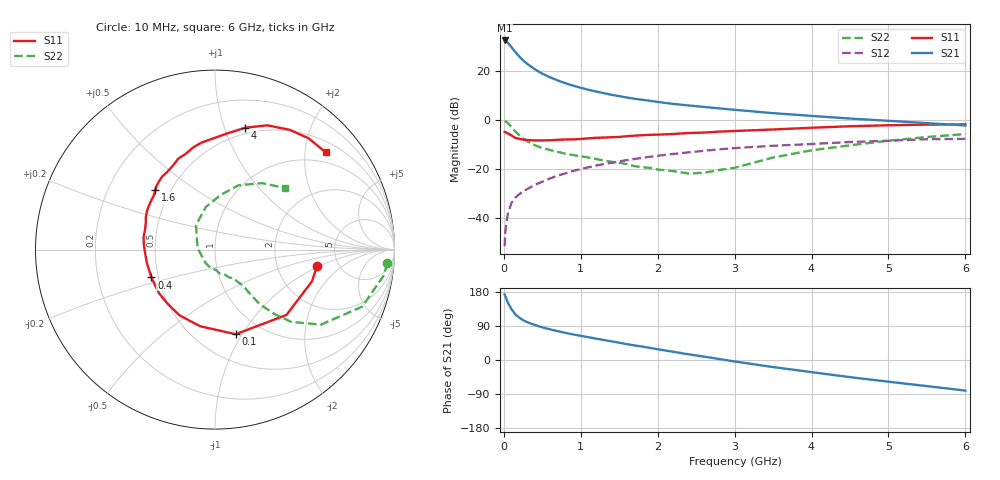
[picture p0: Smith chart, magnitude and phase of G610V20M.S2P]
! SIEMENS Small Signal Semiconductors
! BFG193
! Si NPN RF Bipolar Junction Transistor in SOT223
! VCE = 10 V  IC = 20 mA
! Common Emitter S-Parameters:  August  1996
# GHz  S  MA  R  50
!  f  S11  S21  S12  S22
! GHz  MAG  ANG  MAG  ANG  MAG  ANG  MAG  ANG
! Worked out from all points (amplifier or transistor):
!   36 points, 10 MHz to 6 GHz, reference 50 ohm
!   highest |S21| = 32.5 dB at 10 MHz (marker M1)
!   |S21| within 3 dB of that: start of sweep to 106.1 MHz
!   unconditionally stable (mu >= 1): 743.1 MHz to 2.596 GHz
!   at 250 MHz: K = 0.72, MSG = 26.7 dB, |S12| = -29.1 dB
!   at 1.4 GHz: K = 1.05, MAG = 12.5 dB, |S12| = -17.4 dB
!   at 6 GHz: K = 0.88, MSG = 2.7 dB, |S12| = -7.6 dB
!   S11 on the Smith chart (normalised r, x): 10 MHz: 3.45, -0.92; 100 MHz: 0.76, -0.94; 400 MHz: 0.46, -0.17; 1.6 GHz: 0.41, +0.35; 4 GHz: 0.44, +1.18; 6 GHz: 0.74, +2.46
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0.01  0.5756 -8.9  42.12 173.3  0.0027 89.0  0.9638 -4.5
0.02  0.5687 -18.1  41.56 168.5  0.0054 82.9  0.9491 -9.0
0.05  0.5395 -42.5  38 152.2  0.012 73.4  0.8792 -21.2
0.1  0.4852 -76.3  30.69 134.1  0.0207 64.0  0.7235 -35.3
0.15  0.435 -101.0  24.26 120.1  0.0264 58.6  0.5847 -43.5
0.2  0.4162 -118.4  19.89 111.9  0.0309 58.4  0.4931 -47.1
0.25  0.4007 -131.7  16.58 105.1  0.0352 58.0  0.4214 -49.5
0.3  0.3951 -142.4  14.2 100.2  0.0392 59.1  0.3755 -50.9
0.4  0.3868 -156.4  10.97 92.7  0.0476 59.6  0.3094 -51.7
0.5  0.3868 -168.5  8.856 86.1  0.0557 59.8  0.2699 -51.9
0.6  0.3894 -176.3  7.482 80.9  0.0647 59.9  0.246 -52.8
0.7  0.3969 176.5  6.46 76.1  0.0738 59.9  0.2257 -54.4
0.9  0.4053 164.2  5.058 67.5  0.0922 57.8  0.1942 -56.6
1.1  0.426 154.8  4.162 60.1  0.1095 55.3  0.1732 -63.2
1.6  0.4709 134.9  2.889 41.8  0.1535 46.7  0.1266 -82.3
2.2  0.5222 116.9  2.145 21.8  0.2046 34.4  0.0915 -124.3
2.8  0.5834 101.7  1.735 2.6  0.2543 21.5  0.0964 175.5
3.5  0.6454 85.0  1.39 -18.6  0.3004 5.0  0.1733 127.7
4  0.6998 76.1  1.221 -32.0  0.3261 -4.6  0.2425 102.2
4.5  0.7516 67.1  1.078 -45.3  0.3589 -14.7  0.3067 84.0
5.5  0.8103 49.9  0.87 -68.9  0.4085 -38.1  0.4535 54.8
6  0.8209 41.3  0.78 -80.8  0.4165 -51.7  0.5211 41.1
